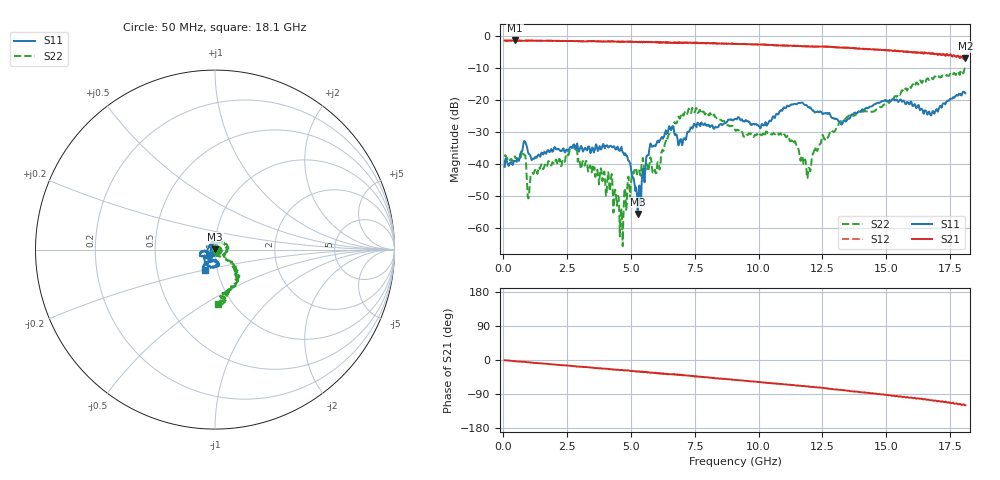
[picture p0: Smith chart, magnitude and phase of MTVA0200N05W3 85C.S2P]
! Network Analyzer HP8720D.06.14 Serial No. US36140669
! 17 Jan 2005  14:03:18
! Frequency  S11  S21  S12  S22
# HZ  S  DB R 50
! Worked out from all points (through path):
!   801 points, 50 MHz to 18.1 GHz, reference 50 ohm
!   highest |S21| = -1.43 dB at 456.1 MHz (marker M1); lowest = -6.9 dB at 18.1 GHz (marker M2)
!   group delay of S21, straight-line fit = 17.5 ps
!   lowest |S11| = -55.7 dB at 5.262 GHz (marker M3), VSWR 1.00, Z = 50 + j0.164 ohm
!   |S11| at or under -10 dB: start of sweep to end of sweep
!   |S22| runs from -65.7 to -10.2 dB; largest |S21 - S12| = 0.027
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5e7  -40.92 -21.5  -1.46 -0.6  -1.46 -1.1  -40.97 -3.6
4.56125e8  -39.05 15.1  -1.43 -3.0  -1.46 -3.3  -37.62 -5.5
7.945625e8  -33.20 25.0  -1.54 -4.9  -1.49 -5.1  -36.88 -42.5
1.020188e9  -36.98 -4.8  -1.47 -6.1  -1.48 -6.4  -48.05 87.8
2.689812e9  -35.02 28.9  -1.57 -15.8  -1.59 -16.1  -35.45 88.2
3.073375e9  -34.87 44.3  -1.66 -18.0  -1.62 -18.3  -40.43 -82.8
4.178938e9  -34.40 4.0  -1.76 -23.7  -1.72 -24.1  -48.57 -134.1
4.630188e9  -34.62 23.2  -1.79 -26.2  -1.80 -26.7  -54.20 -121.5
4.83325e9  -37.59 30.2  -1.78 -27.4  -1.79 -27.6  -53.05 -26.9
5.261938e9  -55.66 84.5  -1.89 -30.4  -1.85 -30.5  -42.37 -56.4
5.690625e9  -37.28 -125.4  -1.89 -31.9  -1.85 -32.6  -42.26 -123.2
6.074188e9  -32.72 -114.9  -2.07 -35.7  -2.06 -35.8  -39.67 134.5
6.615688e9  -28.68 -117.2  -2.14 -37.7  -2.11 -37.8  -28.38 68.1
7.202312e9  -30.07 116.3  -2.07 -41.1  -2.12 -41.7  -24.34 25.7
9.075e9  -26.00 -148.9  -2.55 -52.6  -2.49 -52.9  -29.32 -72.0
1.108306e10  -22.31 -168.6  -3.02 -64.4  -3.05 -64.9  -31.66 -66.5
1.1963e10  -22.29 -151.2  -3.23 -70.3  -3.28 -70.6  -41.22 -13.8
1.209838e10  -23.10 -140.2  -3.28 -71.1  -3.30 -71.3  -37.70 -18.8
1.32265e10  -27.49 -119.1  -3.64 -78.9  -3.63 -79.3  -26.65 -14.3
1.509919e10  -20.37 -109.5  -4.60 -93.1  -4.47 -93.8  -20.92 -41.4
1.670112e10  -24.09 -95.4  -5.43 -105.6  -5.47 -106.9  -13.59 -53.9
1.81e10  -17.93 -114.9  -6.95 -119.6  -6.69 -119.8  -10.28 -87.1
